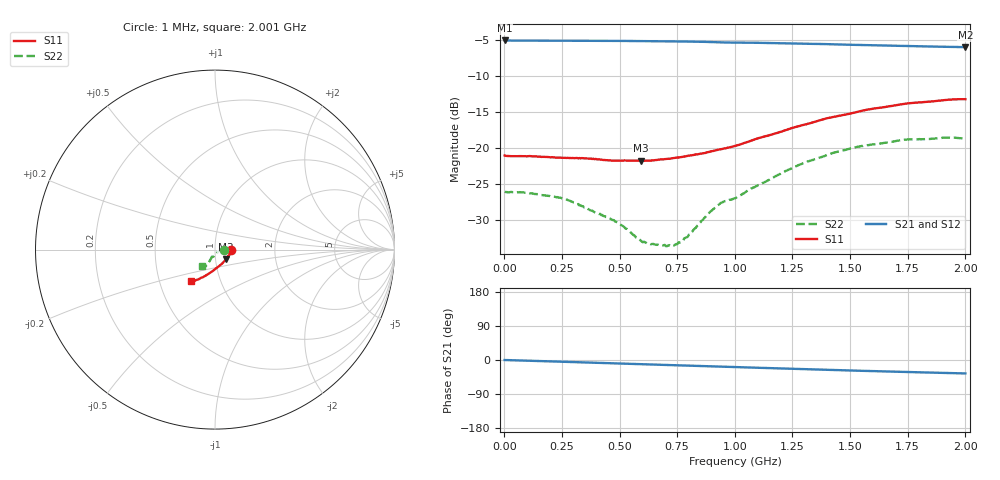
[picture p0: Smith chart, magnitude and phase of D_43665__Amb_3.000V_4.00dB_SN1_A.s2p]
! device id: 43665_
! dir: \\malibu\benchdata\1_engineers\tn_data\43665_75ohm\new\sparar\43665_\amb\3p000v\4p00db
! Serial: 1
! Insertion: A
! Temp: Amb
! VDD: 3.000V
! Attenuation Step: 4.00dB
! IDD: 1.453957e+00mA
! FILE NAME
! DATE 03-27-2009 08:34:21
! CORRECTED  DATA
#  Hz  S  RI  R  75
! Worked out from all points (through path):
!   401 points, 1 MHz to 2.001 GHz, reference 75 ohm
!   highest |S21| = -5.00 dB at 1 MHz (marker M1); lowest = -5.9 dB at 2.001 GHz (marker M2)
!   group delay of S21, straight-line fit = 50.2 ps
!   lowest |S11| = -21.8 dB at 591 MHz (marker M3), VSWR 1.18, Z = 84.2 - j9.22 ohm
!   |S11| at or under -10 dB: start of sweep to end of sweep
!   |S22| runs from -33.7 to -18.5 dB; largest |S21 - S12| = 0.0024
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1000000  0.0887 -0.00129  0.5626 -0.000902  0.5627 -0.000832  0.0496 -0.000425
8.6e7  0.0875 -0.00716  0.5615 -0.0153  0.5617 -0.0153  0.049 0.00116
2.36e8  0.0836 -0.0193  0.5595 -0.0421  0.5598 -0.0423  0.0451 0.00103
3.36e8  0.0802 -0.0286  0.5571 -0.0601  0.5572 -0.0602  0.0394 0.000918
4.81e8  0.0701 -0.0423  0.5521 -0.0861  0.5522 -0.0863  0.0305 -0.00404
5.91e8  0.0607 -0.0544  0.5467 -0.1056  0.5467 -0.1058  0.021 -0.00865
6.26e8  0.0572 -0.0585  0.5449 -0.1116  0.5448 -0.1119  0.0187 -0.011
6.71e8  0.0526 -0.0643  0.5426 -0.1198  0.5425 -0.12  0.0153 -0.0144
7.31e8  0.0461 -0.0714  0.5388 -0.1306  0.5389 -0.1307  0.0106 -0.0182
7.61e8  0.0424 -0.0752  0.5368 -0.136  0.5367 -0.1361  0.00776 -0.0205
8.01e8  0.0376 -0.0802  0.5338 -0.1433  0.5337 -0.1433  0.00374 -0.0246
8.86e8  0.0239 -0.0907  0.5259 -0.1585  0.5259 -0.1584  -0.00376 -0.0348
9.26e8  0.0176 -0.0956  0.521 -0.1646  0.5212 -0.1643  -0.00898 -0.0388
9.51e8  0.0147 -0.098  0.5184 -0.1674  0.5186 -0.1671  -0.0139 -0.04
1.001e9  0.00818 -0.1032  0.5155 -0.1735  0.5157 -0.1734  -0.0183 -0.0406
1.211e9  -0.0274 -0.1289  0.497 -0.2068  0.4977 -0.2071  -0.0287 -0.0616
1.336e9  -0.0487 -0.1425  0.4835 -0.2237  0.4842 -0.2241  -0.0375 -0.0736
1.511e9  -0.0776 -0.1573  0.4637 -0.2454  0.4641 -0.2463  -0.0483 -0.0878
1.671e9  -0.1003 -0.1678  0.4463 -0.2628  0.4458 -0.2641  -0.0564 -0.0944
1.746e9  -0.1099 -0.1723  0.438 -0.2703  0.4376 -0.2718  -0.0602 -0.0977
1.916e9  -0.1263 -0.1758  0.4202 -0.2856  0.4195 -0.2858  -0.0689 -0.0964
2.001e9  -0.1311 -0.1757  0.4119 -0.2929  0.4097 -0.294  -0.0701 -0.0927
